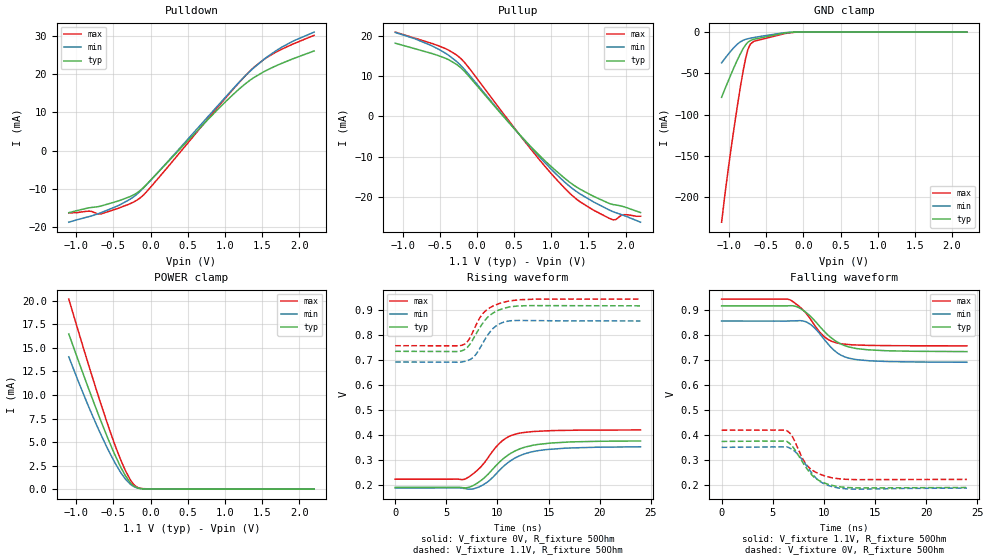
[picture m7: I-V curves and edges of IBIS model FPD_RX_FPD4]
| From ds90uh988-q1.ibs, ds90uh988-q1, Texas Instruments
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|   FPD_RX_FPD4
[Model]   FPD_RX_FPD4
Model_type   I/O
Polarity   Non-Inverting
Enable   Active-High
Vinl = 0
Vinh = 0
Vmeas = 0.55
Vref = 0.55
Cref = 0.02pF
Rref = 50
|   typ   min   max
C_comp   0.838pF   0.838pF   0.878pF
[Voltage Range]   1.1   1.045   1.155
[Temperature Range]   27   105   -40
[Pullup Reference]   1.1   1.045   1.155
[Pulldown Reference]   0   0   0
[Power Clamp Reference]   1.1   1.045   1.155
[GND Clamp Reference]   0   0   0
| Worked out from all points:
|   slope of the pulldown table from 0 to 0.165 V, typ, clamps not added: 49 ohm
|   slope of the pullup table from 0 to 0.165 V, typ, clamps not added: 46.1 ohm
|   GND clamp passes 1 mA (typ) near -0.23 V on its own axis
|   POWER clamp passes 1 mA (typ) near -0.30 V on its own axis
|   falling waveform, V_fixture 1.1V, R_fixture 50Ohm: 20-80 % time 2.83ns typ, 2.26ns min, 2.22ns max; typ from 0.916 V to 0.733 V
|   rising waveform, V_fixture 0V, R_fixture 50Ohm: 20-80 % time 3.19ns typ, 3.06ns min, 2.48ns max; typ from 0.19 V to 0.376 V
|   rising waveform, V_fixture 1.1V, R_fixture 50Ohm: 20-80 % time 1.87ns typ, 1.57ns min, 1.78ns max; typ from 0.734 V to 0.916 V
|   falling waveform, V_fixture 0V, R_fixture 50Ohm: 20-80 % time 1.97ns typ, 1.87ns min, 1.7ns max; typ from 0.374 V to 0.19 V
[Pulldown]
|   Voltage   I(typ)   I(min)   I(max)
-1.1V     -16.14mA   -18.63mA   -16.2mA
-822.8mV  -14.87mA   -17.15mA   -15.76mA
-667.7mV  -14.41mA   -16.15mA   -16.47mA
-413.6mV  -12.96mA   -14.11mA   -14.86mA
-152.9mV  -10.56mA   -10.8mA    -12.48mA
48.4mV    -6.707mA   -6.724mA   -8.425mA
972.4mV   12.07mA    13.19mA    12.91mA
1.203V    16.26mA    18.09mA    18.02mA
1.375V    18.85mA    21.35mA    21.45mA
1.563V    20.97mA    24.36mA    24.27mA
1.754V    22.67mA    26.84mA    26.34mA
2.2V      25.99mA    30.89mA    30.05mA
[GND Clamp]
|   Voltage   I(typ)   I(min)   I(max)
-1.1V     -78.89mA   -37.24mA   -230mA
-1.054V   -68.55mA   -31.73mA   -195.6mA
-977.9mV  -52.09mA   -23.19mA   -144.3mA
-892.1mV  -34.54mA   -14.96mA   -91.9mA
-816.2mV  -20.98mA   -10.18mA   -50mA
-776.6mV  -15.44mA   -8.795mA   -31.83mA
-743.6mV  -12.15mA   -7.988mA   -20.63mA
-710.6mV  -10.12mA   -7.331mA   -14.32mA
-667.7mV  -8.662mA   -6.569mA   -11.24mA
-275mV    -1.521mA   -923.7uA   -2.307mA
-90.2mV   -68.22uA   -53.18uA   -130.3uA
2.2V      0A         0A         0A
[Pullup]
|   Voltage   I(typ)   I(min)   I(max)
-1.1V     18.25mA    20.92mA    21.02mA
-608.3mV  15.69mA    17.61mA    18.2mA
-380.6mV  14.13mA    15.23mA    16.52mA
-228.8mV  12.31mA    12.91mA    14.63mA
-123.2mV  10.31mA    10.76mA    12.46mA
460.9mV   -2.199mA   -2.139mA   -1.863mA
787.6mV   -8.725mA   -9.005mA   -9.587mA
1.111V    -14.32mA   -15.17mA   -16.52mA
1.375V    -17.99mA   -19.16mA   -21.11mA
1.827V    -21.93mA   -23.7mA    -25.73mA
1.976V    -22.5mA    -24.67mA   -24.47mA
2.2V      -23.94mA   -26.34mA   -24.86mA
[POWER Clamp]
|   Voltage   I(typ)   I(min)   I(max)
-1.1V     16.48mA    14.05mA    20.18mA
-971.3mV  13.63mA    11.42mA    16.76mA
-806.3mV  10.09mA    8.26mA     12.49mA
-687.5mV  7.626mA    6.132mA    9.519mA
-502.7mV  4.056mA    3.14mA     5.201mA
-413.6mV  2.533mA    1.915mA    3.343mA
-334.4mV  1.38mA     1.031mA    1.906mA
-255.2mV  541.9uA    422.3uA    793.6uA
-195.8mV  195.9uA    172.9uA    287.9uA
-139.7mV  64.76uA    66.34uA    95.82uA
-44mV     18.37uA    15.34uA    41.21uA
2.2V      0A         0A         0A
[Ramp]
R_load = 50
|   typ   min   max
dV/dt_r   0.111278/3.17657e-09  0.0989202/3.04764e-09   0.11812/2.46914e-09
dV/dt_f   0.109626/2.82252e-09  0.0988168/2.25922e-09   0.112001/2.21445e-09
[Falling Waveform]
V_fixture = 1.1V
V_fixture_min = 1.045V
V_fixture_max = 1.155V
R_fixture = 50Ohm
C_fixture = 0F
|   Time   V(typ)   V(min)   V(max)
0s        915.8mV    855.2mV    942.7mV
6.643ns   916.2mV    855.4mV    940.5mV
7.462ns   910.5mV    856.4mV    917.6mV
8.665ns   875.4mV    842.4mV    864.5mV
9.459ns   840.1mV    811.4mV    818mV
10.08ns   812.3mV    779.8mV    791.6mV
11.5ns    767mV      723mV      765.7mV
12.45ns   751.8mV    706.9mV    761.3mV
14.35ns   740.2mV    696.8mV    758mV
24ns      733.1mV    690.5mV    756mV
[Rising Waveform]
V_fixture = 0V
V_fixture_min = 0V
V_fixture_max = 0V
R_fixture = 50Ohm
C_fixture = 0F
|   Time   V(typ)   V(min)   V(max)
0s        190.2mV    187.5mV    222.8mV
6.861ns   188.1mV    185.1mV    223.8mV
7.658ns   198.2mV    184.4mV    245.6mV
8.587ns   223.7mV    200mV      282mV
9.706ns   270.4mV    237mV      343.9mV
10.4ns    298.3mV    266.3mV    373.5mV
11.14ns   322.1mV    292.3mV    393.8mV
12.06ns   341.8mV    314.3mV    405.9mV
14.75ns   365.2mV    341mV      415.9mV
24ns      375.6mV    352.3mV    419.6mV
[Rising Waveform]
V_fixture = 1.1V
V_fixture_min = 1.045V
V_fixture_max = 1.155V
R_fixture = 50Ohm
C_fixture = 0F
|   Time   V(typ)   V(min)   V(max)
0s        733.9mV    691.3mV    756.2mV
6.643ns   738.1mV    692.4mV    759.9mV
7.148ns   753.9mV    697.8mV    777mV
7.658ns   785.3mV    710.6mV    816.8mV
8.216ns   824.3mV    741.6mV    863.7mV
8.732ns   855mV      778mV      891.3mV
9.719ns   890.3mV    830.4mV    917.7mV
11.13ns   910.7mV    855.1mV    934.8mV
13.67ns   916.5mV    856.6mV    942.3mV
24ns      915.7mV    855.1mV    942.7mV
[Falling Waveform]
|Gnd
V_fixture = 0V
V_fixture_min = 0V
V_fixture_max = 0V
R_fixture = 50Ohm
C_fixture = 0F
|   Time   V(typ)   V(min)   V(max)
0s        374.4mV    350.8mV    419.3mV
6.3ns     375.6mV    352.7mV    419mV
6.92ns    354.7mV    341.9mV    393.7mV
7.914ns   292.1mV    300mV      307.3mV
8.467ns   258.5mV    268.2mV    273.8mV
8.982ns   234.4mV    239.6mV    256.8mV
9.528ns   218.6mV    217.4mV    245.4mV
10.81ns   199.2mV    194mV      229.2mV
13.17ns   189mV      183.8mV    221.9mV
24ns      190.4mV    188mV      222.9mV
